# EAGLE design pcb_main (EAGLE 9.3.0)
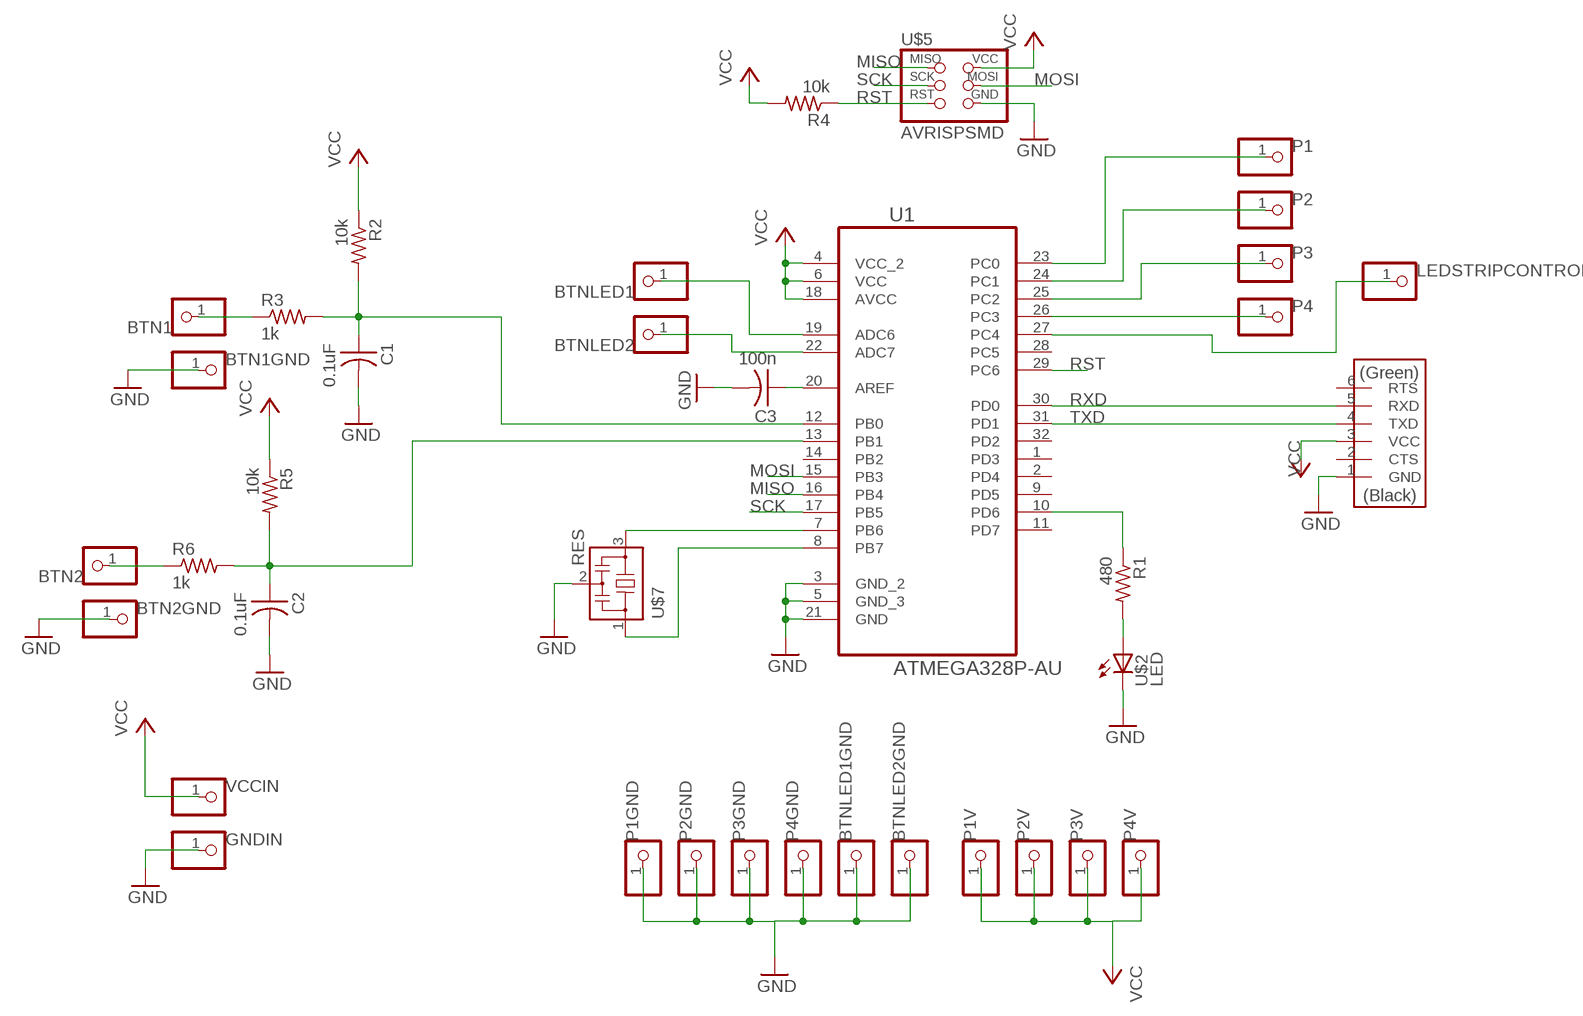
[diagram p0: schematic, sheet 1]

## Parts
BTN1  PINHD-1X1  [1X01]
BTN1GND  PINHD-1X1  [1X01]
BTN2  PINHD-1X1  [1X01]
BTN2GND  PINHD-1X1  [1X01]
BTNLED1  PINHD-1X1  [1X01]
BTNLED1GND  PINHD-1X1  [1X01]
BTNLED2  PINHD-1X1  [1X01]
BTNLED2GND  PINHD-1X1  [1X01]
C1  0.1uF  CAP-US1206FAB  [C1206FAB]
C2  0.1uF  CAP-US1206FAB  [C1206FAB]
C3  100n  CAP-US1206FAB  [C1206FAB]
GNDIN  PINHD-1X1  [1X01]
LEDSTRIPCONTROL  PINHD-1X1  [1X01]
P1  PINHD-1X1  [1X01]
P1GND  PINHD-1X1  [1X01]
P1V  PINHD-1X1  [1X01]
P2  PINHD-1X1  [1X01]
P2GND  PINHD-1X1  [1X01]
P2V  PINHD-1X1  [1X01]
P3  PINHD-1X1  [1X01]
P3GND  PINHD-1X1  [1X01]
P3V  PINHD-1X1  [1X01]
P4  PINHD-1X1  [1X01]
P4GND  PINHD-1X1  [1X01]
P4V  PINHD-1X1  [1X01]
R1  480  RES-US1206FAB  [R1206FAB]
R2  10k  RES-US1206FAB  [R1206FAB]
R3  1k  RES-US1206FAB  [R1206FAB]
R4  10k  RES-US1206FAB  [R1206FAB]
R5  10k  RES-US1206FAB  [R1206FAB]
R6  1k  RES-US1206FAB  [R1206FAB]
U1  ATMEGA328P-AU  [QFP80P900X900X120-32N]
U$1  FTDI-SMD-HEADER  [1X06SMD]
U$2  LED  LEDFAB1206  [LED1206FAB]
U$5  AVRISPSMD  [2X03SMD]
U$7  RES  RESONATOR  [EFOBM]
VCCIN  PINHD-1X1  [1X01]

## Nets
GND: BTN1GND.1 BTN2GND.1 BTNLED1GND.1 BTNLED2GND.1 C1.2 C2.2 C3.2 GNDIN.1 P1GND.1 P2GND.1 P3GND.1 P4GND.1 U1.3(GND_2) U1.5(GND_3) U1.21(GND) U$1.1(GND) U$2.2(C) U$5.6(GND) U$7.2
MISO: U1.16(PB4) U$5.1(MISO)
MOSI: U1.15(PB3) U$5.4(MOSI)
N$1: BTN1.1 R3.1
N$2: P1.1 U1.23(PC0)
N$3: C3.1 U1.20(AREF)
N$4: BTN2.1 R6.1
N$5: R1.1 U1.10(PD6)
N$6: LEDSTRIPCONTROL.1 U1.27(PC4)
N$7: R1.2 U$2.1(A)
N$8: P2.1 U1.24(PC1)
N$9: C1.1 R2.2 R3.2 U1.12(PB0)
N$10: BTNLED1.1 U1.19(ADC6)
N$11: P4.1 U1.26(PC3)
N$12: BTNLED2.1 U1.22(ADC7)
N$13: C2.1 R5.2 R6.2 U1.13(PB1)
N$14: U1.7(PB6) U$7.3
N$15: U1.8(PB7) U$7.1
P3: P3.1 U1.25(PC2)
RST: R4.1 U1.29(PC6) U$5.5(RST)
RXD: U1.30(PD0) U$1.5(RXD)
SCK: U1.17(PB5) U$5.3(SCK)
TXD: U1.31(PD1) U$1.4(TXD)
VCC: P1V.1 P2V.1 P3V.1 P4V.1 R2.1 R4.2 R5.1 U1.4(VCC_2) U1.6(VCC) U1.18(AVCC) U$1.3(VCC) U$5.2(VCC) VCCIN.1
Unconnected: U1.1(PD3) U1.2(PD4) U1.9(PD5) U1.11(PD7) U1.14(PB2) U1.28(PC5) U1.32(PD2) U$1.2(CTS) U$1.6(RTS)

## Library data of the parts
BTN1 BTN1GND BTN2 BTN2GND BTNLED1 BTNLED1GND BTNLED2 BTNLED2GND GNDIN LEDSTRIPCONTROL P1 P1GND P1V P2 P2GND P2V P3 P3GND P3V P4 P4GND P4V VCCIN = pinhead:PINHD-1X1: PIN HEADER
C1-C3 = fab:CAP-US
R1-R6 = fab:RES-US: Resistor (US Symbol)
U1 = Atmel_By_element14_Batch_1-00:ATMEGA328P-AU: 8-bit Microcontroller with In-System Programmable Flash; MPN: ATMEGA328P-AU; OC_FARNELL: 1715486; OC_NEWARK: 14R4631; PACKAGE: TQFP-32; SUPPLIER: Atmel
U$1 = fab:FTDI-SMD-HEADER
U$2 = fab:LED: LED
U$5 = fab:AVRISP
U$7 = fab:RESONATOR

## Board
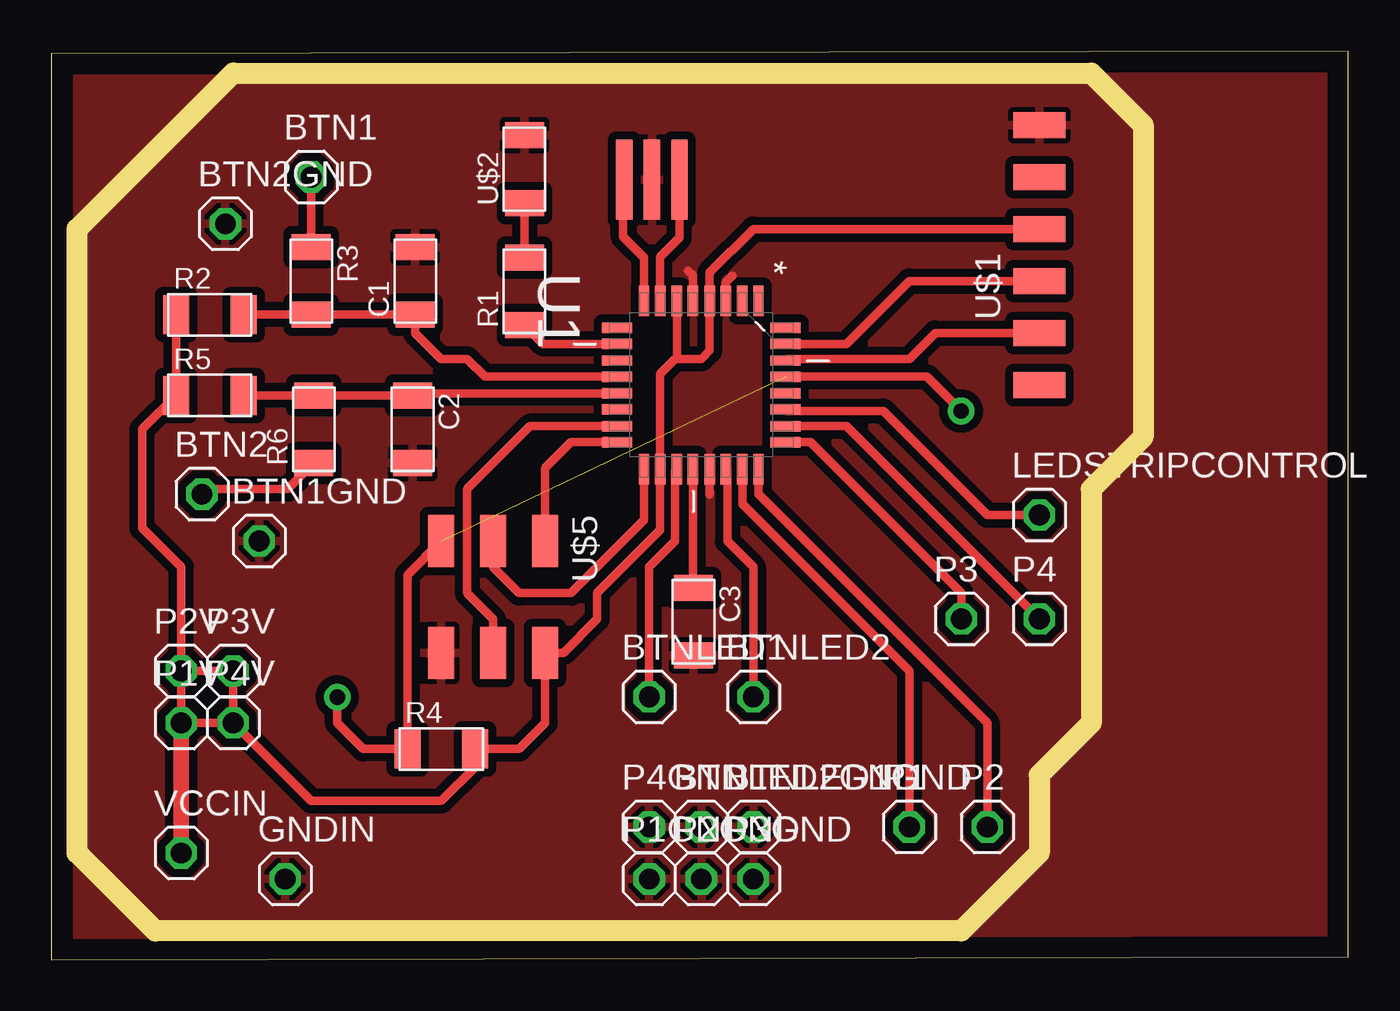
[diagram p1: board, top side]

Size 63.35 x 44.37 mm. Coordinates in mm from the lower left corner, seen from the top.
Outline: 0,0 63.35,0.13 63.35,44.37 0,44.25 0,0
Copper layers (1*16): Top 0.035mm / dielectric 1.5mm / Bottom 0.035mm
Design rules "default *": minimum track width 16mil, minimum drill 0.35mm, track to track 16mil, track to pad 14mil, pad to pad 10mil, via to via 16mil, smd to smd 16mil, copper to edge 40mil, drill to drill 6mil, minimum pad ring 10mil, minimum via ring 8mil, stop-mask expansion 4mil, vias tented up to drill 0mil, thermal gap 10mil
Milling: 14 lines

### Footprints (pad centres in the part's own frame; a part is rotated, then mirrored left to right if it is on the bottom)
1X01 = drill 1.016 octagon: 1 0,0
C1206FAB = smd 1.27 x 1.905: 1 -1.651,0; 2 1.651,0
R1206FAB = smd 1.27 x 1.905: 1 -1.651,0; 2 1.651,0
QFP80P900X900X120-32N = smd 1.473 x 0.508: 1 -4.115,2.794; 2 -4.115,2.007; 3 -4.115,1.194; 4 -4.115,0.406; 5 -4.115,-0.406; 6 -4.115,-1.194; 7 -4.115,-2.007; 8 -4.115,-2.794; 17 4.115,-2.794; 18 4.115,-2.007; 19 4.115,-1.194; 20 4.115,-0.406; 21 4.115,0.406; 22 4.115,1.194; 23 4.115,2.007; 24 4.115,2.794 | smd 0.508 x 1.473: 9 -2.794,-4.115; 10 -2.007,-4.115; 11 -1.194,-4.115; 12 -0.406,-4.115; 13 0.406,-4.115; 14 1.194,-4.115; 15 2.007,-4.115; 16 2.794,-4.115; 25 2.794,4.115; 26 2.007,4.115; 27 1.194,4.115; 28 0.406,4.115; 29 -0.406,4.115; 30 -1.194,4.115; 31 -2.007,4.115; 32 -2.794,4.115
1X06SMD = smd 2.54 x 1.27: 1 0,6.35; 2 0,3.81; 3 0,1.27; 4 0,-1.27; 5 0,-3.81; 6 0,-6.35
LED1206FAB = smd 1.27 x 1.905: 1 -1.651,0; 2 1.651,0
2X03SMD = smd 2.54 x 1.27: 1 -2.54,2.54; 2 2.92,2.54; 3 -2.54,0; 4 2.92,0; 5 -2.54,-2.54; 6 2.92,-2.54
EFOBM = smd 0.8 x 3.9: 1 -1.35,0; 2 0,0; 3 1.35,0

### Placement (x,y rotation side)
BTN1  12.7,38.23 0 top
BTN1GND  10.16,20.45 0 top
BTN2  7.37,22.73 0 top
BTN2GND  8.51,35.94 0 top
BTNLED1  29.21,12.83 0 top
BTNLED1GND  34.29,6.48 0 top
BTNLED2  34.29,12.83 0 top
BTNLED2GND  31.75,6.48 0 top
C1  17.78,33.15 90 top
C2  17.65,25.91 270 top
C3  31.37,16.51 270 top
GNDIN  11.43,3.94 0 top
LEDSTRIPCONTROL  48.26,21.72 0 top
P1  41.91,6.48 0 top
P1GND  29.21,3.94 0 top
P1V  6.35,11.56 0 top
P2  45.72,6.48 0 top
P2GND  31.75,3.94 0 top
P2V  6.35,14.1 0 top
P3  44.45,16.64 0 top
P3GND  34.29,3.94 0 top
P3V  8.89,14.1 0 top
P4  48.26,16.64 0 top
P4GND  29.21,6.48 0 top
P4V  8.89,11.56 0 top
R1  23.11,32.64 90 top
R2  7.75,31.5 0 top
R3  12.7,33.15 270 top
R4  19.05,10.29 0 top
R5  7.75,27.56 0 top
R6  12.83,25.91 90 top
U1  31.75,28.07 270 top
U$1  48.26,34.42 0 top
U$2  23.11,38.61 90 top
U$5  21.59,17.91 270 top
U$7  29.34,38.1 0 top
VCCIN  6.35,5.21 0 top

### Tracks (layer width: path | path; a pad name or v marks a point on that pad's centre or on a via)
GND
  Top 0.406: U1.21 32.16,22.71 | U1.3 32.94,33.07 33.27,33.4 | U1.5 31.34,33.43 31.11,33.66
  pour Top: 1.27,43.31 1.27,0.13 62.23,0.13 62.23,43.31
MISO
  Top 0.406: U1.16 25.4,25.27 24.13,24 U$5.1
MOSI
  Top 0.406: U1.15 23.39,26.06 20.32,22.99 20.32,17.91 21.59,16.64 U$5.4
N$1
  Top 0.406: R3.1 BTN1.1
N$2
  Top 0.406: U1.23 33.76,22.25 41.91,14.1 P1.1
N$3
  Top 0.406: U1.20 31.34,18.19 C3.1
N$4
  Top 0.406: R6.1 11.56,22.99 7.62,22.99 BTN2.1
N$5
  Top 0.406: U1.10 24.03,30.07 R1.1
N$6
  Top 0.406: U1.27 35.94,26.8 40.64,26.8 45.72,21.72 LEDSTRIPCONTROL.1
N$7
  Top 0.406: U$2.1 R1.2
N$8
  Top 0.406: U1.24 34.54,22.73 45.72,11.56 P2.1
N$9
  Top 0.406: U1.12 21.18,28.47 20.32,29.34 19.05,29.34 17.78,30.61 C1.1 R3.2 R2.2
N$10
  Top 0.406: U1.19 30.48,23.88 30.48,20.45 29.21,19.18 BTNLED1.1
N$11
  Top 0.406: U1.26 38.84,26.06 P4.1
N$12
  Top 0.406: U1.22 33.02,23.88 33.02,20.45 34.29,19.18 BTNLED2.1
N$13
  Top 0.406: U1.13 17.76,27.66 C2.1 R6.2 R5.2
N$14
  Top 0.406: U1.7 29.74,34.31 30.69,35.26 U$7.3
N$15
  Top 0.406: U1.8 28.96,34.29 27.94,35.31 27.94,38.05 U$7.1
N$16  (via drill 0.75 pad 1.3)
  other vias: 44.45,26.8
P3
  Top 0.406: P3.1 44.45,17.91 37.08,25.27 U1.25
RST  (via drill 0.75 pad 1.3)  (1 unrouted)
  Top 0.406: U$5.5 17.4,18.8 R4.1 15.24,10.29 13.97,11.56 v13.97,12.83 | U1.29 42.77,28.47 44.45,26.8
RXD
  Top 0.406: U1.30 35.94,29.34 41.91,29.34 43.18,30.61 U$1.5
SCK
  Top 0.406: U1.17 28.96,21.46 25.4,17.91 22.86,17.91 21.59,19.18 U$5.3
TXD
  Top 0.406: U1.31 38.84,30.07 41.91,33.15 U$1.4
VCC
  Top 0.406: U$1.3 34.29,35.69 32.16,33.55 U1.4 32.16,29.74 31.75,29.34 30.48,29.34 | P4V.1 P1V.1 P2V.1 | P4V.1 P3V.1 P2V.1 | P4V.1 12.7,7.75 19.05,7.75 20.7,9.4 R4.2 22.86,10.29 24.13,11.56 U$5.2 25.02,14.99 26.67,16.64 26.67,17.91 29.74,20.98 U1.18 29.74,28.6 30.48,29.34 | P2V.1 6.35,19.18 4.45,21.08 4.45,25.91 R5.1 R2.1 | U1.6 30.56,29.41 30.48,29.34
  Top 0.762: VCCIN.1 P1V.1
